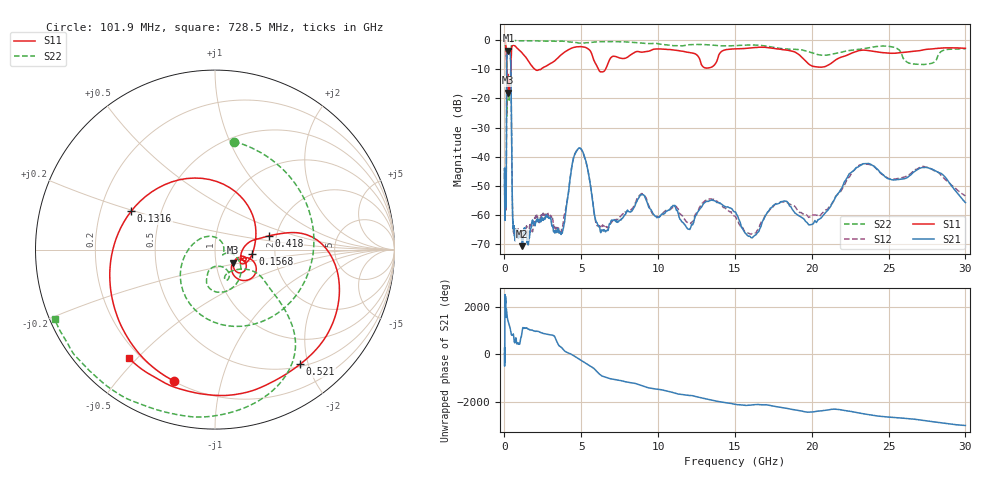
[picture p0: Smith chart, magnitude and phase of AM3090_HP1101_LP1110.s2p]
! Date/Time: Thu, Feb 28, 2019 2:08 PM
! Network Analyzer: Agilent Technologies E8364B Rev: A.07.50.67
! Sweep from 0.010 to 30.000 GHz, 1601 Points, Sweep Type: LOG
! Power Supply: 5.022 V, 0.002 A
# Hz S DB R 50
!freq MagS11 AngS11 MagS21 AngS21 MagS12 AngS12 MagS22 AngS22
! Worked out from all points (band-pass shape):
!   1601 points, 10 MHz to 30 GHz, reference 50 ohm
!   highest |S21| = -3.66 dB at 262.5 MHz (marker M1); lowest = -70.6 dB at 1.154 GHz (marker M2)
!   |S21| within 3 dB of the highest: 154.7 MHz to 400.3 MHz (245.7 MHz wide, 88.5 % of centre)
!   lowest |S11| = -18.1 dB at 249.7 MHz (marker M3), VSWR 1.29, Z = 60.6 - j8.87 ohm
!   |S11| at or under -10 dB: 144.1 MHz to 419.4 MHz (275.3 MHz wide, 97.7 % of centre); 1.971 GHz to 2.385 GHz (413.8 MHz wide, 19 % of centre); 6.109 GHz to 6.584 GHz (475.1 MHz wide, 7.49 % of centre)
!   |S22| runs from -26.1 to -0.2 dB; largest |S21 - S12| = 0.013
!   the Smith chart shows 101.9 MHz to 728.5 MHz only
!   S11 on the Smith chart (normalised r, x): 101.9 MHz: 0.20, -0.71; 131.6 MHz: 0.33, +0.19; 156.8 MHz: 1.52, -0.07; 418 MHz: 1.82, +0.31; 521 MHz: 0.54, -1.87; 728.5 MHz: 0.16, -0.47
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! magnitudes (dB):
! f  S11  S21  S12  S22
! 10 MHz  -0.3  -47.6  -47.6  -0.7
! 38.04 MHz  -0.3  -56.6  -57.4  -1.5
! 101.9 MHz  -2.3  -53.3  -56.4  -4.3
! 115 MHz  -3.3  -54.8  -54.0  -4.9
! 131.6 MHz  -5.8  -30.5  -30.9  -6.4
! 144.7 MHz  -10.3  -11.8  -11.7  -16.7
! 156.8 MHz  -13.6  -6.2  -6.2  -26.0
! 249.7 MHz  -18.1  -3.7  -3.6  -14.7
! 262.5 MHz  -16.5  -3.7  -3.6  -15.8
! 418 MHz  -10.2  -9.8  -9.8  -7.0
! 521 MHz  -2.0  -57.3  -57.3  -0.5
! 550.5 MHz  -1.9  -62.1  -64.0  -0.4
! 728.5 MHz  -2.2  -66.2  -66.4  -0.2
! 1.154 GHz  -4.5  -70.6  -66.7  -0.3
! 2.084 GHz  -10.4  -61.7  -59.9  -0.3
! 3.704 GHz  -5.0  -66.1  -65.4  -0.4
! 4.878 GHz  -2.3  -37.0  -37.0  -1.1
! 6.171 GHz  -10.6  -64.1  -63.6  -0.6
! 7.926 GHz  -6.1  -58.9  -59.2  -0.7
! 16.05 GHz  -2.7  -67.7  -66.5  -1.7
! 23.48 GHz  -3.5  -42.3  -42.4  -2.9
! 30 GHz  -2.9  -55.7  -53.4  -3.0
